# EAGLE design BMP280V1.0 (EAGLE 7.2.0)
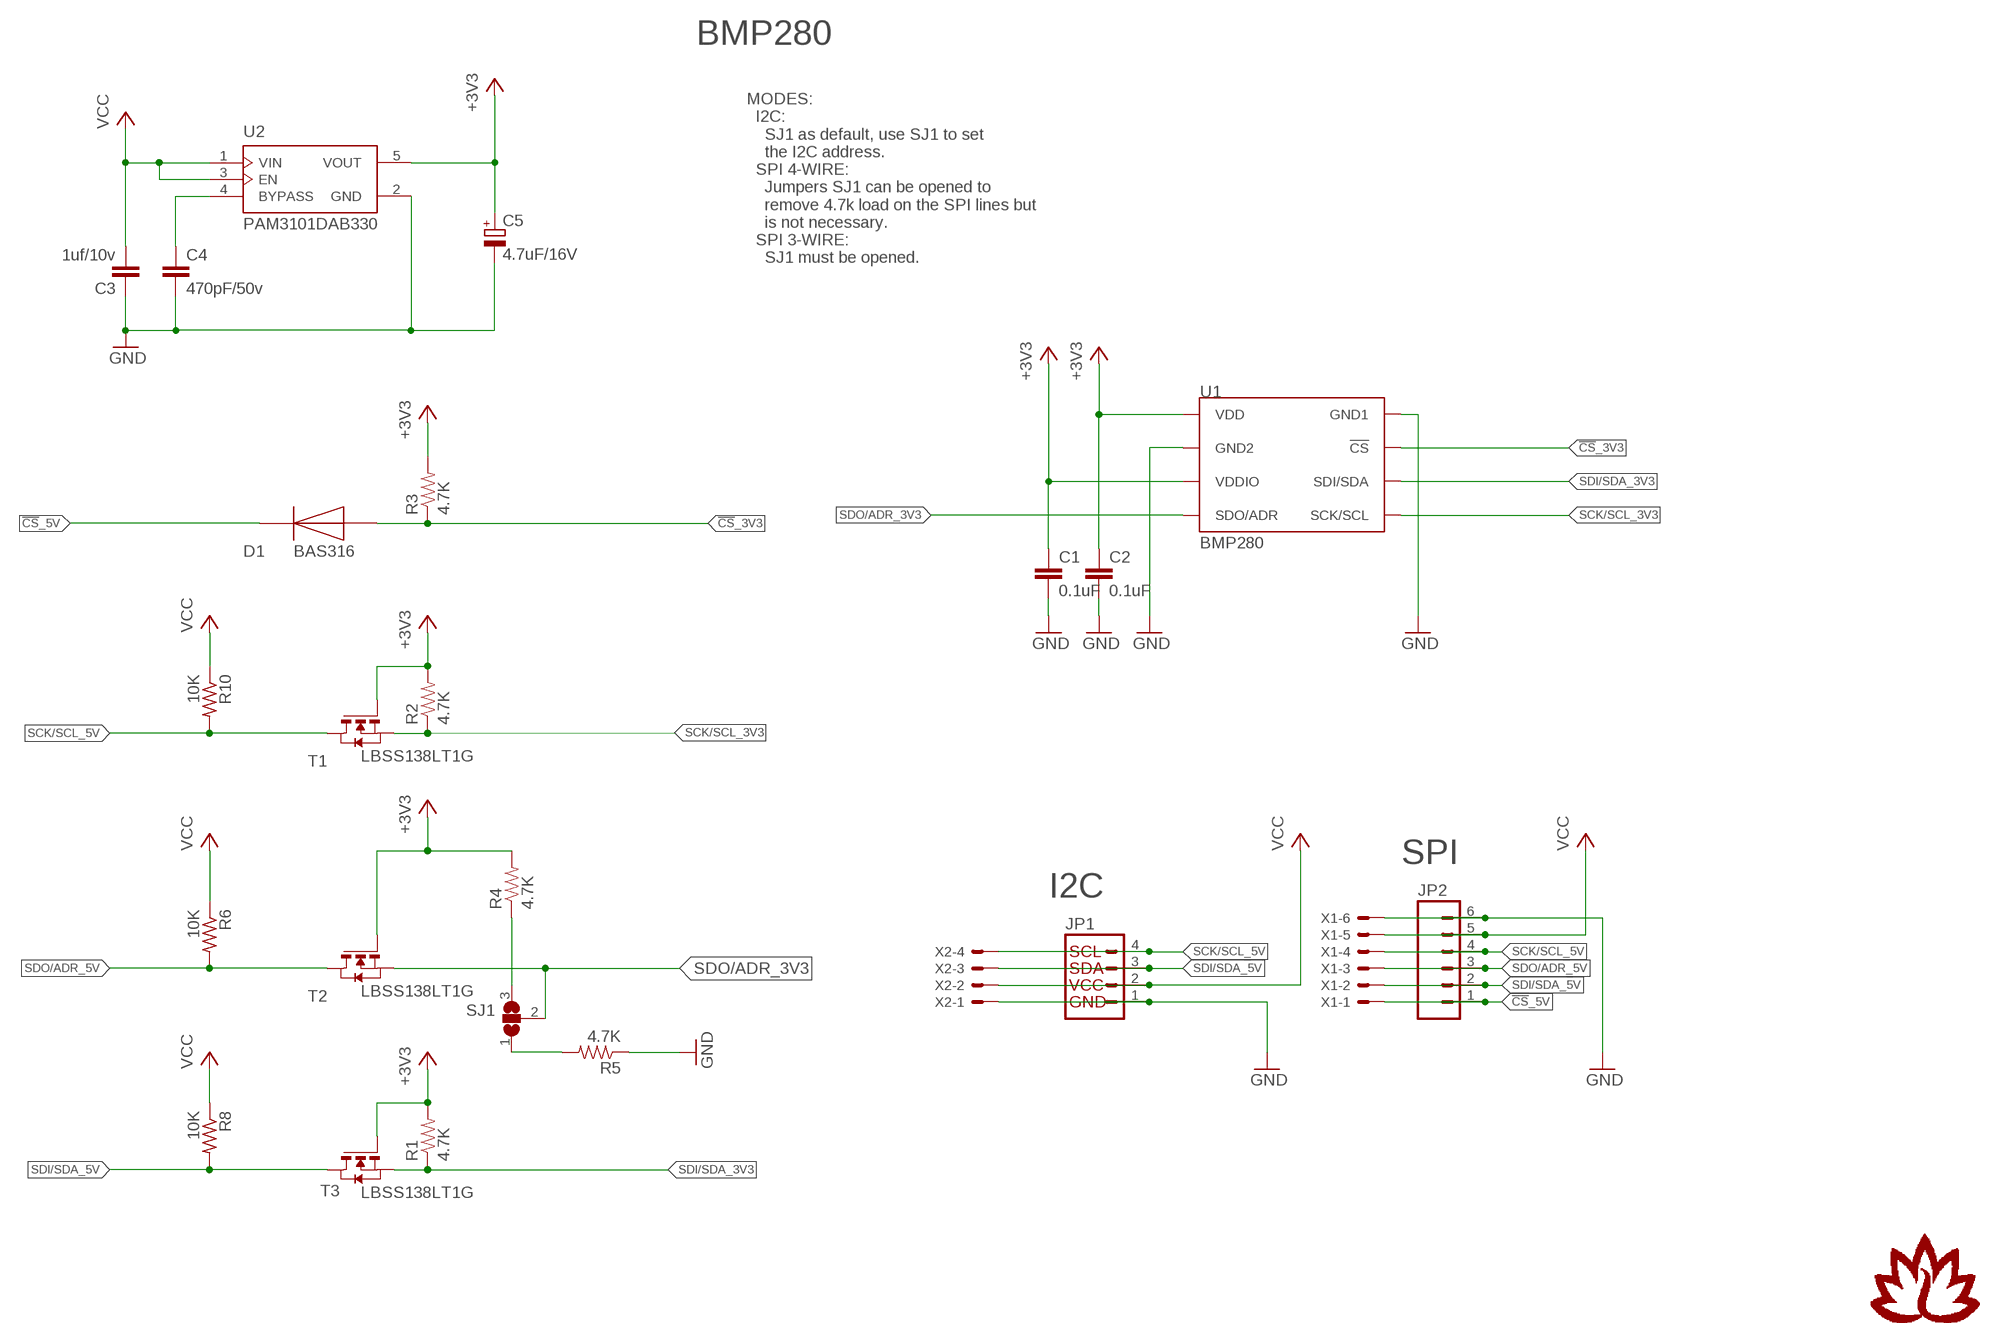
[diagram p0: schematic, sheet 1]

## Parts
C1  0.1uF  0.1UF-25V-5%(0603)  [0603-CAP]
C2  0.1uF  0.1UF-25V-5%(0603)  [0603-CAP]
C3  1uf/10v  C-EUC0603  [C0603]
C4  470pF/50v  C-EUC0603  [C0603]
C5  4.7uF/16V  CPOL-EUA/3216-18R  [A/3216-18R]
D1  BAS316  [SOD323_ST]
JP1  I2C_STANDARD_NO_SILK  [1X04_NO_SILK]
JP2  M06NO_SILK_FEMALE_PTH  [1X06_NO_SILK]
R1  4.7K  4.7KOHM-1/10W-1%(0603)  [0603-RES]
R2  4.7K  4.7KOHM-1/10W-1%(0603)  [0603-RES]
R3  4.7K  4.7KOHM-1/10W-1%(0603)  [0603-RES]
R4  4.7K  4.7KOHM-1/10W-1%(0603)  [0603-RES]
R5  4.7K  4.7KOHM-1/10W-1%(0603)  [0603-RES]
R6  10K  R-US_R0603  [R0603]
R8  10K  R-US_R0603  [R0603]
R10  10K  R-US_R0603  [R0603]
SJ1  EN ADR PULLUP  SJ2W  [SJ_2]
T1  LBSS138LT1G  NMOSSOT23  [SOT-23]
T2  LBSS138LT1G  NMOSSOT23  [SOT-23]
T3  LBSS138LT1G  NMOSSOT23  [SOT-23]
U1  BMP280  [BMP280]
U2  PAM3101DAB330  [SOT23-5]
X1  53261-06  [53261-06]
X2  53261-04  [53261-04]

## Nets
!CS!_3V3: D1.A R3.1 U1.2(!CS)
!CS!_5V: D1.C(K) JP2.1 X1.1
+3V3: C1.1 C2.1 C5.+ R1.2 R2.2 R3.2 R4.2 T1.3(G) T2.3(G) T3.3(G) U1.6(VDDIO) U1.8(VDD) U2.5(VOUT)
GND: C1.2 C2.2 C3.1 C4.2 C5.- JP1.1 JP2.6 R5.1 U1.1(GND1) U1.7(GND2) U2.2(GND) X1.6 X2.1
N$1: R4.1 SJ1.3
N$2: R5.2 SJ1.1
N$6: C4.1 U2.4(BYPASS)
SCK/SCL_3V3: R2.1 T1.2(S) U1.4(SCK/SCL)
SCK/SCL_5V: JP1.4 JP2.4 R10.2 T1.1(D) X1.4 X2.4
SDI/SDA_3V3: R1.1 T3.2(S) U1.3(SDI/SDA)
SDI/SDA_5V: JP1.3 JP2.2 R8.2 T3.1(D) X1.2 X2.3
SDO/ADR_3V3: SJ1.2 T2.2(S) U1.5(SDO/ADR)
SDO/ADR_5V: JP2.3 R6.2 T2.1(D) X1.3
VCC: C3.2 JP1.2 JP2.5 R6.1 R8.1 R10.1 U2.1(VIN) U2.3(EN) X1.5 X2.2

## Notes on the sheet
- BMP280
- MODES:
    I2C:
      SJ1 as default, use SJ1 to set
      the I2C address.
    SPI 4-WIRE:
      Jumpers SJ1 can be opened to 
      remove 4.7k load on the SPI lines but
      is not necessary.
    SPI 3-WIRE:
      SJ1 must be opened.
- SPI
- I2C

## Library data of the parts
C1 C2 = SparkFun-Capacitors:0.1UF-25V-5%(0603): CAP-08604; PROD_ID: CAP-08604
C3 C4 = rcl:C-EU: CAPACITOR, European symbol
C5 = rcl:CPOL-EU: POLARIZED CAPACITOR, European symbol
D1 = cus:BAS316
JP1 = SparkFun-Connectors:I2C_STANDARD: SparkFun has standardized on a pinout for all I2C based sensor breakouts. This pinout allows I2C boards to be plugged directly into the headers on Arduino Uno compatible boards, and to be daisy chained easily.
JP2 = SparkFun-Connectors:M06: Header 6 Standard 6-pin 0.1" header. Use with straight break away headers (SKU : PRT-00116), right angle break away headers (PRT-00553), swiss pins (PRT-00743), machine pins (PRT-00117), and female headers (PRT-00115). Molex polarized connector foot print use with SKU : PRT-08094 with associated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; PROD_ID: CONN-08437
R1-R5 = SparkFun-Resistors:4.7KOHM-1/10W-1%(0603): RES-07857; PROD_ID: RES-07857
R6 R8 R10 = rcl:R-US_: RESISTOR, American symbol
SJ1 = jumper:SJ2W: SMD solder JUMPER
T1-T3 = zetex:NMOSSOT23: MOS FET; OC_FARNELL: unknown; OC_NEWARK: unknown
U1 = BMP280:BMP280
U2 = cus:PAM3101DAB330
X1 = con-molex:53?-06: CONNECTOR wire to board 1.25 mm (.049 inch) pitch header; OC_FARNELL: 1125375; OC_NEWARK: unknown
X2 = con-molex:53?-04: CONNECTOR wire to board 1.25 mm (.049 inch) pitch header; OC_FARNELL: 1125374; OC_NEWARK: unknown

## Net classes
0 default: clearance 0.205 mm

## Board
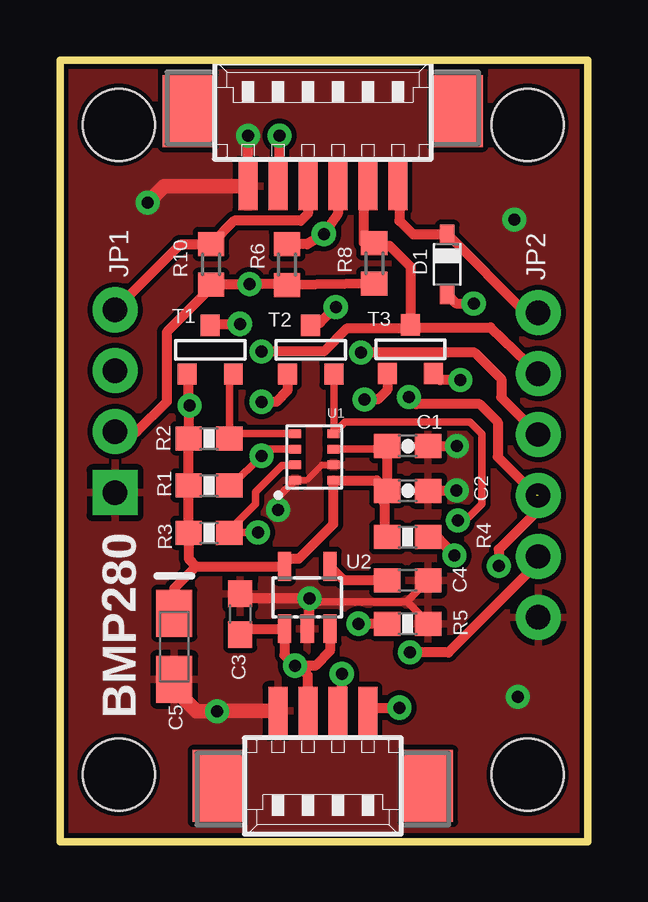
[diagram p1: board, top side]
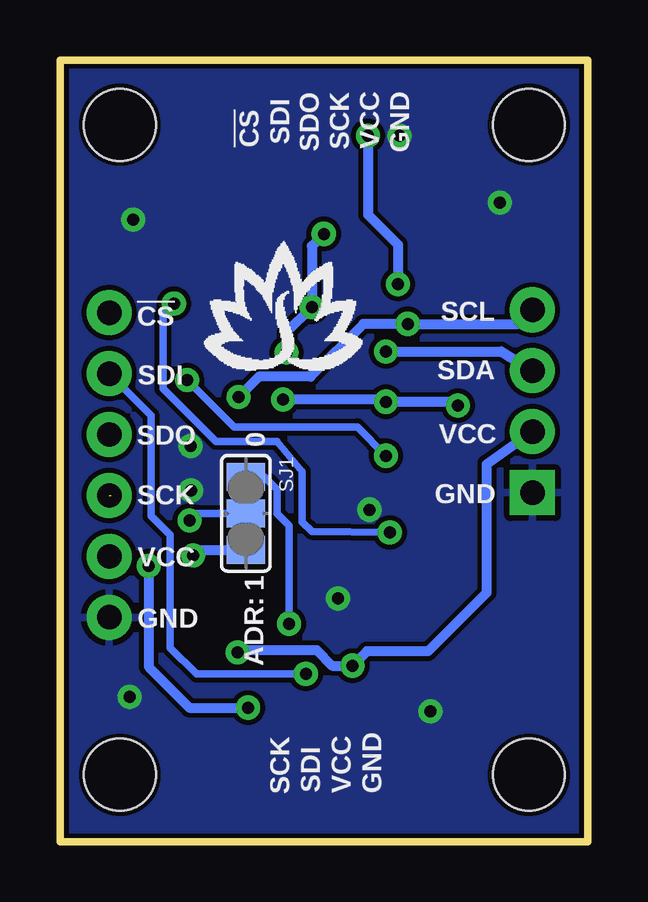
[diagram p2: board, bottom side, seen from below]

Size 22 x 32.6 mm. Coordinates in mm from the lower left corner, seen from the top.
Outline: 0,32.6 22,32.6 22,0 0,0 0,32.6
Copper layers (1*16): Top 0.035mm / dielectric 1.5mm / Bottom 0.035mm
Design rules "SparkFun-2-layer *": minimum track width 7mil, minimum drill 15mil, track to track 8mil, track to pad 8mil, pad to pad 8mil, via to via 8mil, smd to smd 8mil, copper to edge 8mil, drill to drill 8mil, minimum pad ring 10mil, minimum via ring 10mil, stop-mask expansion 4mil, vias tented up to drill 20mil, thermal gap 10mil
Holes 3 mm at 2.45,2.8 19.5,2.8 19.5,29.9 2.45,29.9

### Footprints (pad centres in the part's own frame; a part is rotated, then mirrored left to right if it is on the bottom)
0603-CAP = smd 1.1 x 1: 1 -0.85,0; 2 0.85,0
C0603 = smd 1.1 x 1: 1 -0.85,0; 2 0.85,0
A/3216-18R = smd 1.95 x 1.5: + 1.375,0; - -1.375,0
SOD323_ST = smd 0.8 x 0.6: A 1.25,0; C -1.25,0
1X04_NO_SILK = drill 1.016 pad 1.88 square: 1 0,0 | drill 1.016 pad 1.88: 2 2.54,0; 3 5.08,0; 4 7.62,0
1X06_NO_SILK = drill 1.016 pad 1.88: 1 0,0; 2 2.54,0; 3 5.08,0; 4 7.62,0; 5 10.16,0; 6 12.7,0
0603-RES = smd 1.1 x 1: 1 -0.85,0; 2 0.85,0
R0603 = smd 1 x 1.1: 1 -0.85,0; 2 0.85,0
SJ_2 = smd 1.168 x 1.6: 1 -1.524,0; 2 0,0; 3 1.524,0
SOT-23 = smd 0.787 x 0.889: 1 0.025,-1.016; 2 -0.94,1.016; 3 0.991,1.016
BMP280 = smd 0.5 x 0.35: 1 0.8,0.975; 2 0.8,0.325; 3 0.8,-0.325; 4 0.8,-0.975; 5 -0.8,-0.975; 6 -0.8,-0.325; 7 -0.8,0.325; 8 -0.8,0.975
SOT23-5 = smd 0.55 x 1.2: 1 -0.95,-1.3; 2 0,-1.3; 3 0.95,-1.3; 4 0.95,1.3; 5 -0.95,1.3
53261-06 = smd 0.8 x 2: 1 3.125,-2.5; 2 1.875,-2.5; 3 0.625,-2.5; 4 -0.625,-2.5; 5 -1.875,-2.5; 6 -3.125,-2.5 | smd 2.1 x 3: S1 5.625,0.625; S2 -5.625,0.625
53261-04 = smd 0.8 x 2: 1 1.875,-2.5; 2 0.625,-2.5; 3 -0.625,-2.5; 4 -1.875,-2.5 | smd 2.1 x 3: S1 4.375,0.625; S2 -4.375,0.625

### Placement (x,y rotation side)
C1  14.5,16.5 0 top
C2  14.5,14.64 0 top
C3  7.52,9.5 270 top
C4  14.5,10.91 0 top
C5  4.77,8.15 90 top
D1  16.15,24.08 270 top
JP1  2.29,14.56 90 top
JP2  19.94,22.06 270 top
R1  6.22,14.86 180 top
R2  6.22,16.82 180 top
R3  6.22,12.89 180 top
R4  14.5,12.71 180 top
R5  14.5,9.1 180 top
R6  9.47,24.07 90 top
R8  13.11,24.12 90 top
R10  6.3,24.08 90 top
SJ1  14.25,13.7 270 bottom
T1  6.29,20.52 180 top
T2  10.48,20.52 180 top
T3  14.64,20.54 180 top
U1  10.6,16.05 180 top
U2  10.31,10.19 0 top
X1  10.96,29.84 0 top
X2  10.96,2.96 180 top

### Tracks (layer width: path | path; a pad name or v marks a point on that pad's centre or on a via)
!CS!_3V3  (via drill 0.5)
  Top 0.305: 7.35,13.17 R3.1 | R3.1 7.11,12.85 7.16,12.9 v8.25,12.9 | R3.1 7.07,13.02 8.15,14.1 8.15,14.6 9.25,15.7 9.78,15.7 U1.2
  Top 0.406: D1.A 16.53,22.45 v17.25,22.45
  Bottom 0.305: v17.25,22.45 17.7,22 17.7,18.9 15.5,16.7 12.95,16.7 11.9,15.45 11.9,13.35 11.5,12.95 v8.25,12.9
!CS!_5V
  Top 0.406: 16.1,25.33 D1.C | D1.C 19.42,22.06 JP2.1 | X1.1 14.15,27.34 14.15,25.9 14.72,25.33 D1.C
+3V3  (via drill 0.5)
  Top 0.305: U1.6 13.52,16.38 arc90 C1.1
  Top 0.406: T1.3 5.35,19.4 5.35,18.25 v5.4,18.2 5.37,16.98 R2.2 R1.2 | R1.2 R3.2 5.37,11.81 5.68,11.49 | R1.2 | T2.3 9.49,18.81 9.03,18.35 v8.4,18.35 | 13.53,14.14 C2.1 | T3.3 13.65,18.85 13.25,18.45 v12.7,18.45 | 13.53,14.14 13.53,12.96 R4.2 | C2.1 C1.1 | 13.49,14.18 13.53,14.14 | 5.68,11.49 U2.5 arc-90 9.67,11.8 9.95,11.8 11.4,13.25 U1.8 13.21,15.08 C2.1 | 5.68,11.49 4.77,10.57 C5.+
  Bottom 0.406: v12.7,18.45 8.5,18.45 v8.4,18.35 5.55,18.35 v5.4,18.2
GND  (via drill 0.5, 0.5 pad 0.25)
  Top 0.254: U1.1 9.82,15.1 10.3,15.1 10.93,15.72 U1.7
  Top 0.305: C4.2 14.47,10.03 | 14.47,10.03 14.44,10 10.55,10 v10.4,10.15 | R5.1 15.35,9.15 14.47,10.03 | U1.1 9.1,14.37 v9.1,13.85
  Top 0.406: X1.6 7.84,29.44 | v7.85,29.45 7.85,29.4 | C1.2 v16.55,16.5 | 15.66,14.65 v16.54,14.65 | U2.2 10.4,8.89 v10.4,10.15 7.72,10.15 C3.1
  Top 0.61: X1.6 4.34,27.34 v3.65,26.65 | X2.1 v6.56,5.46 v6.55,5.45 5.7,5.45 4.77,6.38 C5.-
  other vias: 19.1,6.05 18.95,25.95
  pour Top: 0,32.6 0,0 22,0 22,32.6
  pour Bottom: 0,32.6 0,0 22,0 22,32.6
N$1  (via drill 0.5)
  Top 0.406: R4.1 15.74,12.71 v16.45,11.95
  Bottom 0.406: v16.45,11.95 16.22,12.18 SJ1.3
N$2  (via drill 0.5)
  Top 0.406: R5.2 v12.45,9.1
  Bottom 0.305: v12.45,9.1 12.45,13.2 12.95,13.7 12.95,14.7 13.47,15.22 SJ1.1
N$6
  Top 0.406: C4.1 11.84,10.91 U2.4
SCK/SCL_3V3
  Top 0.305: T1.2 7.07,19.19 R2.1 | 7.09,16.85 R2.1 | U1.4 7.27,17.02 arc90 R2.1
SCK/SCL_5V  (via drill 0.5)  (1 unrouted)
  Top 0.406: X1.4 10.34,26.19 10.05,25.9 7.27,25.9 R10.2 6.27,24.9 5.01,24.9 JP1.4 | T1.1 6.32,21.48 6.43,21.6 v7.5,21.6 | X2.4 12.84,5.6 v14.15,5.6 | 19.86,14.44 18.25,16.05 18.25,17.5 17.5,18.25 14.85,18.25 v14.55,18.55 | JP2.4 19.94,13.84 18.3,12.2 v18.3,11.5
  Bottom 0.406: v14.15,5.6 16.6,5.6 18.3,7.3 v18.3,11.5 | JP1.4 2.88,21.6 v7.5,21.6 9.35,21.6 11.55,19.4 13.7,19.4 v14.55,18.55
SDI/SDA_3V3  (via drill 0.5)
  Top 0.305: 7.07,15.22 R1.1 7.16,14.86 v8.4,16.1 8.68,16.38 U1.3
  Top 0.406: v16.7,19.25 15.85,19.25 T3.2
  Bottom 0.305: v16.7,19.25 14.75,17.3 9.6,17.3 v8.4,16.1
SDI/SDA_5V  (via drill 0.5)
  Top 0.406: X1.2 12.66,27.16 12.66,24.97 R8.2 13.23,24.85 13.75,24.85 14.62,23.98 T3.1 14.64,21.56 14.7,21.5 | 14.7,21.5 14.75,21.45 17.96,21.45 JP2.2 | 14.7,21.5 14.6,21.4 11.95,21.4 11,20.45 v8.4,20.45 | X2.3 11.75,5.62 v11.75,7
  Bottom 0.305: JP2.2 18.2,17.78 18.2,13.6 17.4,12.8 17.4,8.1 16.3,7 v11.75,7
  Bottom 0.406: v8.4,20.45 3.6,20.45 JP1.3
SDO/ADR_3V3  (via drill 0.5)
  Top 0.305: v16.6,13.4 16.9,13.4 17.6,14.1 17.6,17 17.1,17.5 11.88,17.5 U1.5 11.42,17.05 T2.2
  Bottom 0.305: v16.6,13.4 16.3,13.7 SJ1.2
SDO/ADR_5V  (via drill 0.5)
  Top 0.406: X1.3 11.59,26.19 v11,25.35 10.32,24.92 R6.2 | T2.1 10.34,21.65 10.85,21.65 v11.5,22.3 | JP2.3 18.4,18.53 18.4,19.3 17.3,20.4 v12.55,20.4
  Bottom 0.406: v12.55,20.4 12.55,21.25 v11.5,22.3 11.5,24.85 v11,25.35
VCC  (via drill 0.5)
  Top 0.406: R8.1 R6.1 | R6.1 | R10.1 6.35,23.18 | 6.35,23.18 6.35,23.15 4.45,21.25 4.45,18.35 3.2,17.1 JP1.2 | X1.5 9.15,27.4 v9.15,29.45 | 6.35,23.18 6.42,23.25 v7.9,23.25 9.44,23.25 R6.1 | X2.2 10.34,6.96 v9.8,7.35 | v14.6,7.9 16.2,7.9 19.94,11.64 JP2.5 | U2.3 11.26,7.96 10.65,7.35 v9.8,7.35 | v9.8,7.35 9.36,7.79 U2.1 7.6,8.89 7.6,8.5 7.52,8.58 C3.2
  Bottom 0.406: v9.15,29.45 9.15,26.15 7.9,24.9 v7.9,23.25 | JP1.2 4.2,15.75 4.2,10.4 6.65,7.95 9.2,7.95 v9.8,7.35 10.65,7.35 11.3,8 14.5,8 v14.6,7.9

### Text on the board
tPlace: BMP280
bPlace: GND | VCC | SCK | SDO | SDI | !CS | SCL | !CS | SDA | SDI | VCC | SDO | 0 | GND | SCK | VCC | 1 | ADR: | GND | GND | VCC | SDI | SCK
